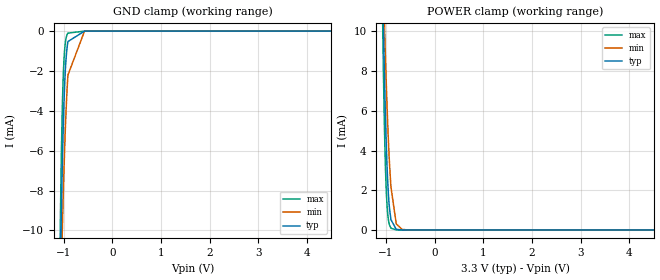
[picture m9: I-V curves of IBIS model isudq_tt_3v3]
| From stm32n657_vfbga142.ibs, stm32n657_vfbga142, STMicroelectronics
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[Model]   isudq_tt_3v3
Model_type Input
Polarity   Non-Inverting
Enable   Active-Low
| CAP_THRESHOLD on pad IOTT is "UDTCAPC" :
| Rising=30.0% of vddiov33m   Falling=70.0% of vddiov33m
| C_comp min and max val. don't necessarily correlate with the min and max pvt
| but are the smallest and greatest pad capacitance found.
| var   typ   min   max
C_comp   1.02819pF  1.02008pF  1.03746pF
|C_comp_pullup   494.67500fF  500.82000fF  492.80000fF
|C_comp_pulldown   533.51008fF  519.26020fF  544.65507fF
Vinl = 1.35V
Vinh = 1.8V
[Model Spec]
| TIME_THRESHOLD on pin ZIV08M is "CMOS" :
| Rising=50.0% of vddv08m   Falling=50.0% of vddv08m
Vinl 1.06670V 940.70000mV 1.19570V
Vinh 1.29530V 1.04830V 1.42630V
| variable   typ   min   max
[Temperature Range] 25.0 125.0 -40.0
| variable   typ   min   max
[Voltage Range] 3.3V 2.7V 3.6V
| variable   typ   min   max
[POWER Clamp Reference] 3.3V 2.7V 3.6V
| variable   typ   min   max
[GND Clamp Reference] 0V 0V 0V
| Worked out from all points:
|   GND clamp passes 1 mA (typ) near -0.94 V on its own axis
|   POWER clamp passes 1 mA (typ) near -0.93 V on its own axis
[POWER Clamp]
-3.3V     566.9mA    322.9mA    1.076A
-1.07V    12.25mA    13.82mA    10.53mA
-1.06V    10.95mA    12.86mA    8.87mA
-1.05V    9.71mA     11.93mA    7.356mA
-1.03V    7.448mA    10.14mA    4.814mA
-1V       4.655mA    7.704mA    2.244mA
-980mV    3.229mA    6.259mA    1.253mA
-950mV    1.728mA    4.398mA    485.7uA
-900mV    522.1uA    2.17mA     91.84uA
-790mV    29.1uA     304.7uA    2.706uA
-670mV    1.316uA    28.48uA    495nA
6.6V      0A         0A         0A
[GND Clamp]
-3.3V     -662mA     -392.1mA   -1.188A
-1.07V    -12.6mA    -14.73mA   -10.39mA
-1.05V    -9.719mA   -12.51mA   -6.951mA
-1.03V    -7.219mA   -10.44mA   -4.332mA
-1.02V    -6.123mA   -9.473mA   -3.329mA
-1V       -4.261mA   -7.674mA   -1.875mA
-980mV    -2.837mA   -6.075mA   -1.005mA
-960mV    -1.813mA   -4.693mA   -523uA
-940mV    -1.121mA   -3.534mA   -269.1uA
-910mV    -523.4uA   -2.205mA   -101.1uA
-570mV    -2.455uA   -5.073uA   -2.525uA
6.6V      44.36nA    287.9nA    5.823nA
